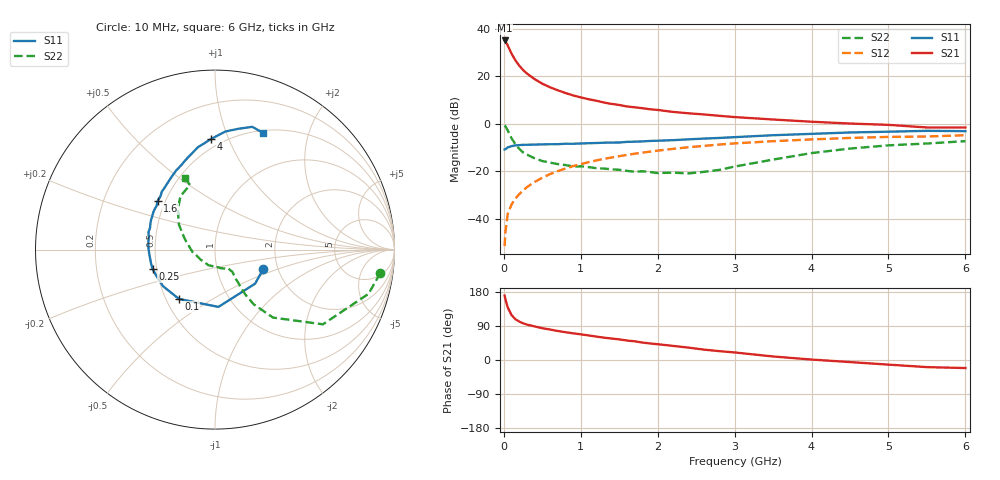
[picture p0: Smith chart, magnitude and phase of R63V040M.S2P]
! SIEMENS Small Signal Semiconductors
! BFR193
! Si NPN RF Bipolar Junction Transistor in SOT23
! VCE = 3 V  IC = 40 mA
! Common Emitter S-Parameters:  May  1996
# GHz  S  MA  R  50
!  f  S11  S21  S12  S22
! GHz  MAG  ANG  MAG  ANG  MAG  ANG  MAG  ANG
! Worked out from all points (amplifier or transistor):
!   36 points, 10 MHz to 6 GHz, reference 50 ohm
!   highest |S21| = 35.1 dB at 10 MHz (marker M1)
!   |S21| within 3 dB of that: start of sweep to 63.52 MHz
!   unconditionally stable (mu >= 1): 408.5 MHz to 1.884 GHz
!   at 250 MHz: K = 0.94, MSG = 25.3 dB, |S12| = -28.0 dB
!   at 1.4 GHz: K = 1.02, MAG = 10.3 dB, |S12| = -14.1 dB
!   at 6 GHz: K = 0.95, MSG = 1.6 dB, |S12| = -4.8 dB
!   S11 on the Smith chart (normalised r, x): 10 MHz: 1.68, -0.39; 100 MHz: 0.58, -0.36; 250 MHz: 0.47, -0.12; 1.6 GHz: 0.45, +0.30; 4 GHz: 0.44, +0.87; 6 GHz: 0.52, +1.35
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0.01  0.2906 -21.6  56.57 170.1  0.0027 87.0  0.9301 -8.1
0.02  0.2931 -40.4  54.38 160.9  0.0053 80.6  0.8901 -16.1
0.05  0.3199 -86.6  44.62 138.9  0.0127 70.1  0.7314 -34.7
0.1  0.3403 -126.1  29.93 118.7  0.0203 67.5  0.4981 -49.5
0.15  0.3543 -144.9  21.63 107.7  0.027 67.9  0.3745 -54.7
0.2  0.3573 -155.3  16.76 101.4  0.0334 70.6  0.3002 -56.0
0.25  0.364 -162.9  13.54 96.9  0.0399 71.2  0.2522 -55.8
0.3  0.3646 -167.3  11.45 93.5  0.0468 72.6  0.2263 -54.9
0.4  0.3669 -176.0  8.716 88.6  0.0603 73.5  0.1891 -54.5
0.5  0.3716 178.1  6.98 83.9  0.0738 73.8  0.1657 -52.5
0.6  0.3735 173.5  5.881 80.4  0.0881 73.1  0.1539 -52.1
0.8  0.3832 165.3  4.461 73.4  0.1155 71.2  0.1365 -54.0
0.9  0.3819 161.2  3.964 70.4  0.1296 70.0  0.1276 -55.1
1.1  0.3925 155.2  3.302 64.9  0.1567 67.6  0.1237 -60.2
1.3  0.4025 148.3  2.814 59.0  0.1842 65.0  0.1153 -66.3
1.6  0.4192 139.8  2.323 51.4  0.2229 60.7  0.1031 -77.5
2.2  0.4551 125.6  1.784 37.2  0.299 51.7  0.0946 -112.9
3.5  0.5781 99.5  1.236 9.3  0.4333 31.2  0.178 160.8
4  0.6173 91.9  1.11 1.2  0.4721 24.2  0.2438 145.4
4.5  0.6604 85.0  1.018 -5.5  0.507 17.0  0.3035 133.1
5.5  0.7148 73.1  0.841 -18.8  0.5431 3.2  0.3869 111.1
6  0.7038 67.8  0.84 -21.2  0.5781 -0.8  0.4338 112.9
